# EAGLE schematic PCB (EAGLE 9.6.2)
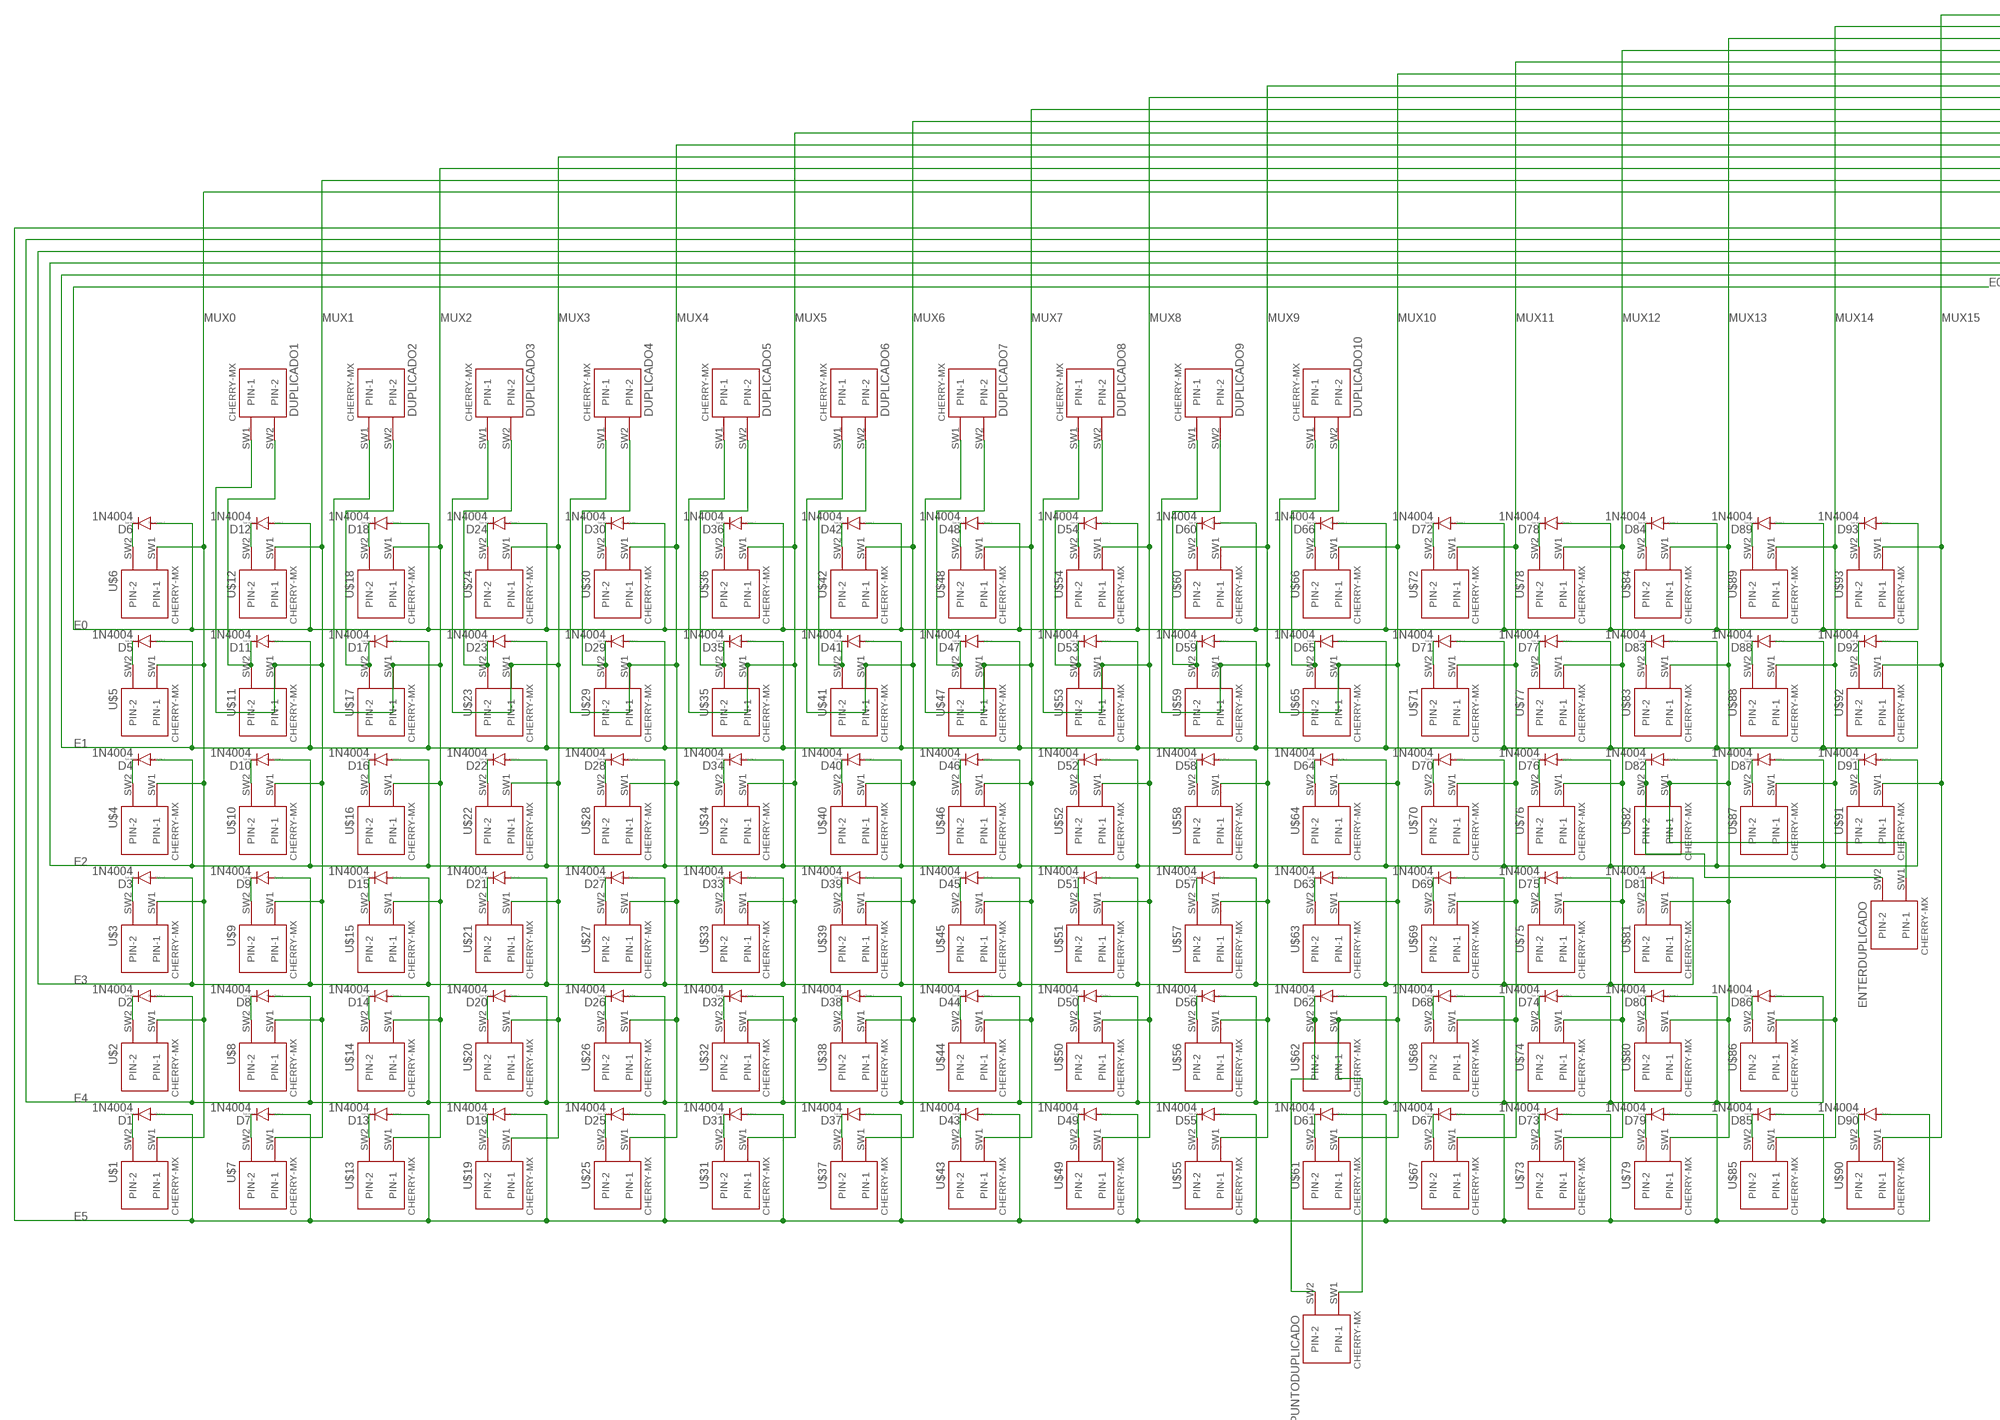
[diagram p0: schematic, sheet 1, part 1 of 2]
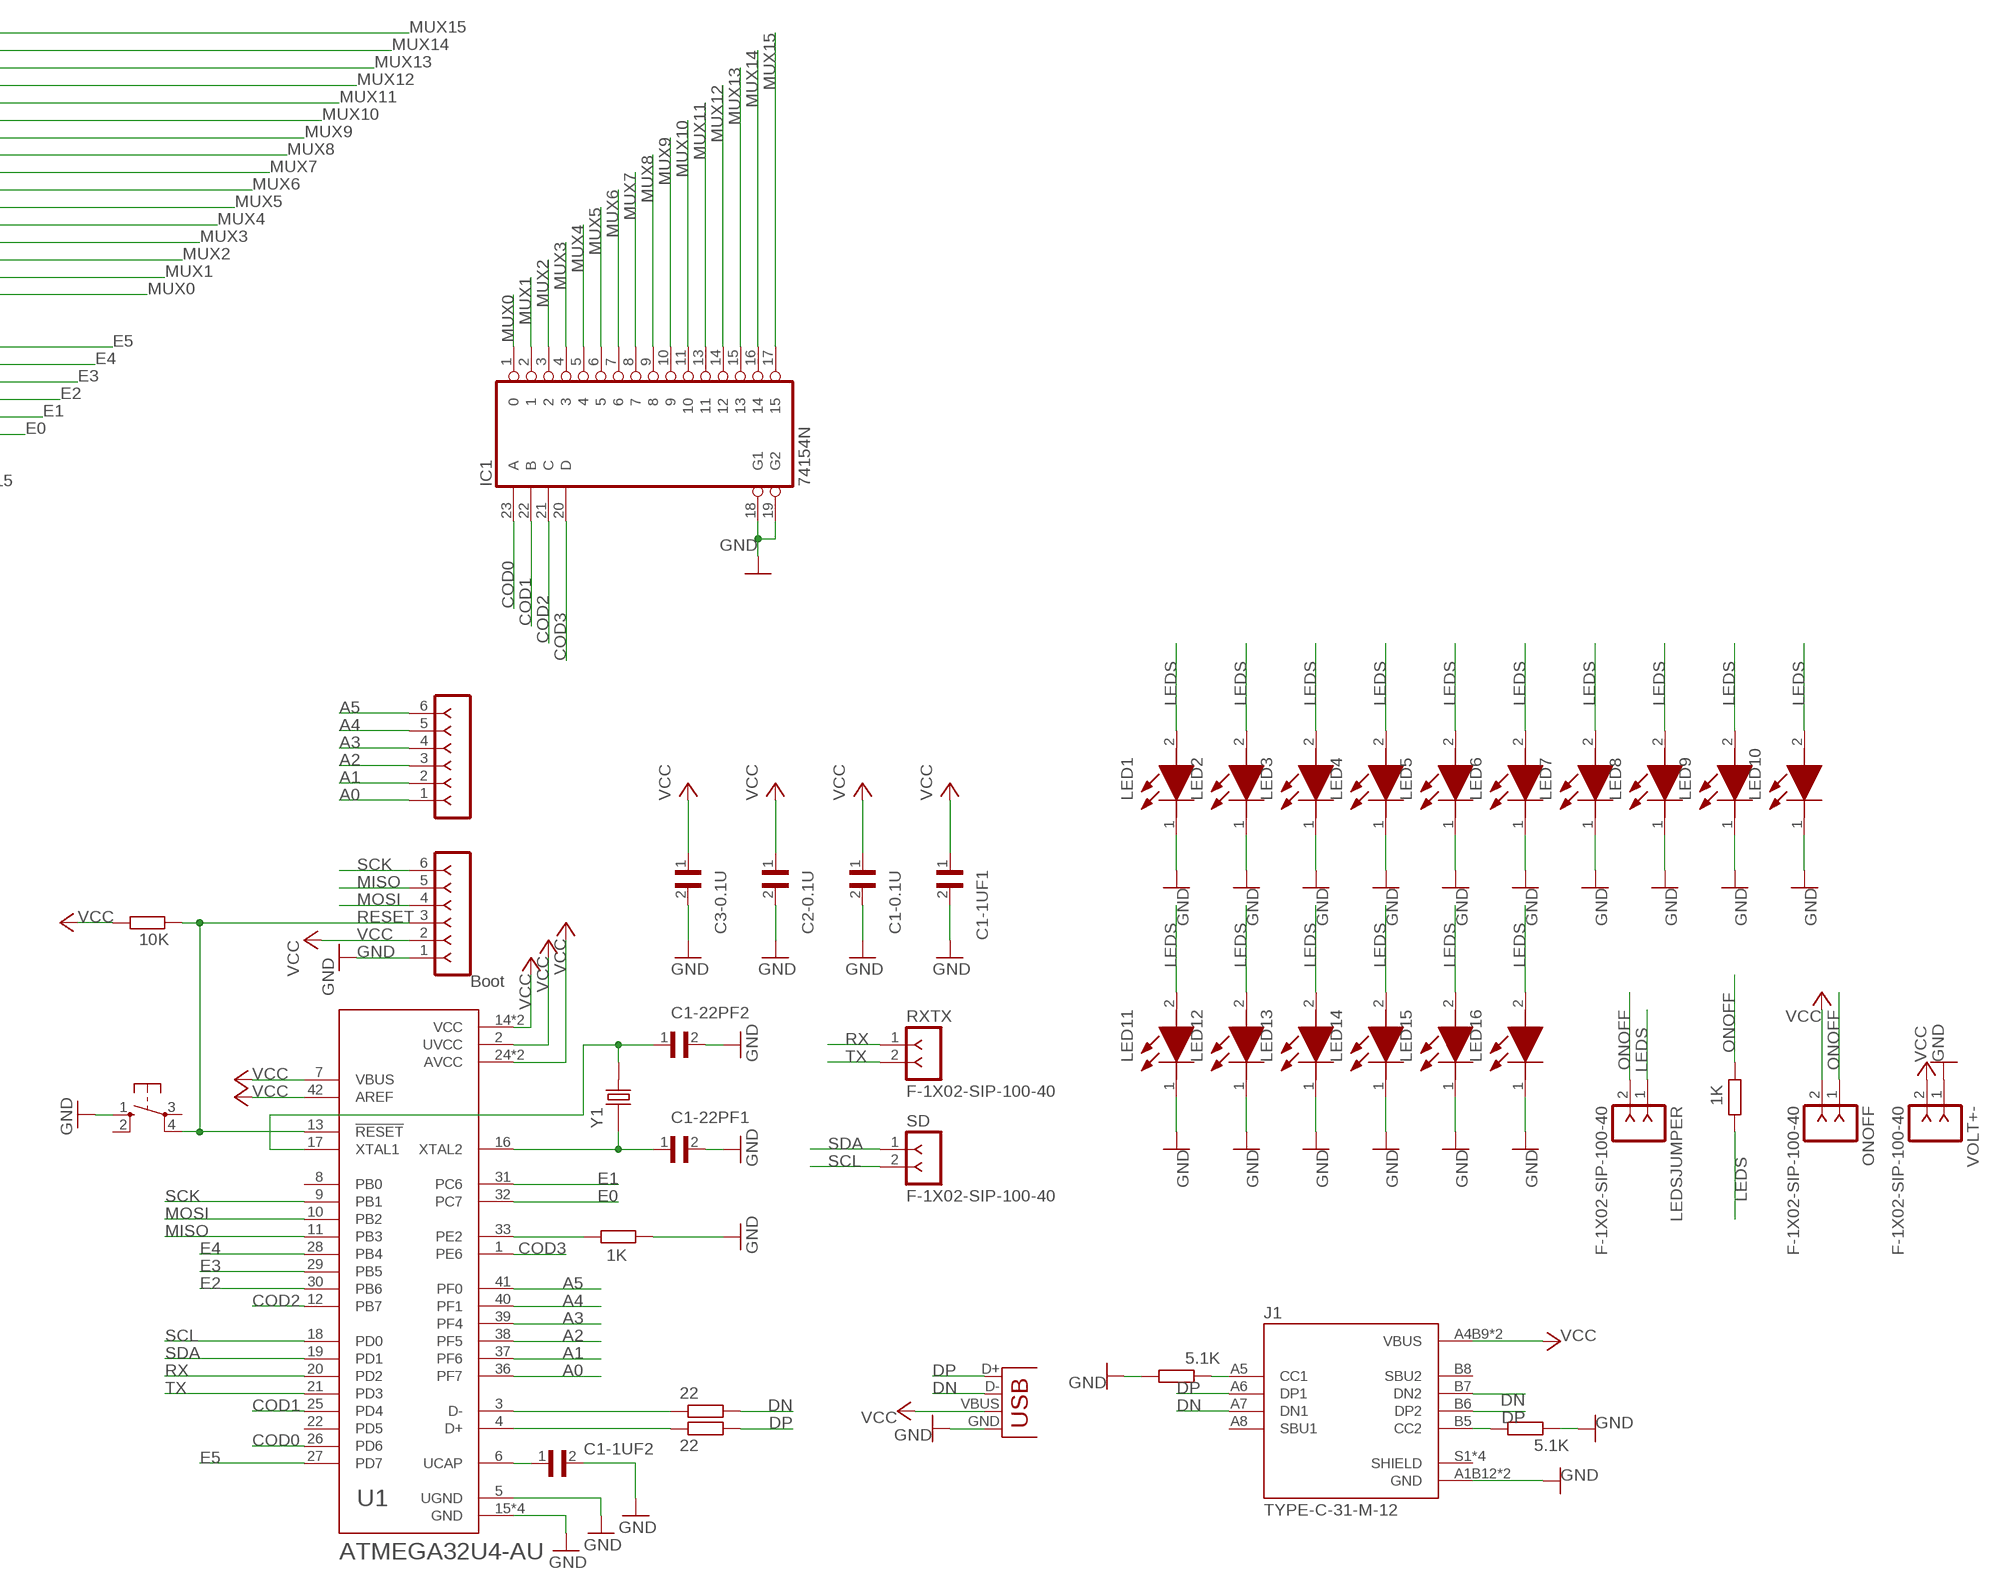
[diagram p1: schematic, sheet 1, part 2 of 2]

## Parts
ANALOG  Boot  F-1X06-SIP-100-32  [SIP-100-06-32]
BUTTON  10-XX  [B3F-10XX]
C1-0.1U  RDE5C1H273J2M1H03A  [CAP_RDE5C1H273J2M1H03A]
C1-1UF1  RDE5C1H273J2M1H03A  [CAP_RDE5C1H273J2M1H03A]
C1-1UF2  RDE5C1H273J2M1H03A  [CAP_RDE5C1H273J2M1H03A]
C1-22PF1  RDE5C1H273J2M1H03A  [CAP_RDE5C1H273J2M1H03A]
C1-22PF2  RDE5C1H273J2M1H03A  [CAP_RDE5C1H273J2M1H03A]
C2-0.1U  RDE5C1H273J2M1H03A  [CAP_RDE5C1H273J2M1H03A]
C3-0.1U  RDE5C1H273J2M1H03A  [CAP_RDE5C1H273J2M1H03A]
D1  1N4004  [DO41-10]
D2  1N4004  [DO41-10]
D3  1N4004  [DO41-10]
D4  1N4004  [DO41-10]
D5  1N4004  [DO41-10]
D6  1N4004  [DO41-10]
D7  1N4004  [DO41-10]
D8  1N4004  [DO41-10]
D9  1N4004  [DO41-10]
D10  1N4004  [DO41-10]
D11  1N4004  [DO41-10]
D12  1N4004  [DO41-10]
D13  1N4004  [DO41-10]
D14  1N4004  [DO41-10]
D15  1N4004  [DO41-10]
D16  1N4004  [DO41-10]
D17  1N4004  [DO41-10]
D18  1N4004  [DO41-10]
D19  1N4004  [DO41-10]
D20  1N4004  [DO41-10]
D21  1N4004  [DO41-10]
D22  1N4004  [DO41-10]
D23  1N4004  [DO41-10]
D24  1N4004  [DO41-10]
D25  1N4004  [DO41-10]
D26  1N4004  [DO41-10]
D27  1N4004  [DO41-10]
D28  1N4004  [DO41-10]
D29  1N4004  [DO41-10]
D30  1N4004  [DO41-10]
D31  1N4004  [DO41-10]
D32  1N4004  [DO41-10]
D33  1N4004  [DO41-10]
D34  1N4004  [DO41-10]
D35  1N4004  [DO41-10]
D36  1N4004  [DO41-10]
D37  1N4004  [DO41-10]
D38  1N4004  [DO41-10]
D39  1N4004  [DO41-10]
D40  1N4004  [DO41-10]
D41  1N4004  [DO41-10]
D42  1N4004  [DO41-10]
D43  1N4004  [DO41-10]
D44  1N4004  [DO41-10]
D45  1N4004  [DO41-10]
D46  1N4004  [DO41-10]
D47  1N4004  [DO41-10]
D48  1N4004  [DO41-10]
D49  1N4004  [DO41-10]
D50  1N4004  [DO41-10]
D51  1N4004  [DO41-10]
D52  1N4004  [DO41-10]
D53  1N4004  [DO41-10]
D54  1N4004  [DO41-10]
D55  1N4004  [DO41-10]
D56  1N4004  [DO41-10]
D57  1N4004  [DO41-10]
D58  1N4004  [DO41-10]
D59  1N4004  [DO41-10]
D60  1N4004  [DO41-10]
D61  1N4004  [DO41-10]
D62  1N4004  [DO41-10]
D63  1N4004  [DO41-10]
D64  1N4004  [DO41-10]
D65  1N4004  [DO41-10]
D66  1N4004  [DO41-10]
D67  1N4004  [DO41-10]
D68  1N4004  [DO41-10]
D69  1N4004  [DO41-10]
D70  1N4004  [DO41-10]
D71  1N4004  [DO41-10]
D72  1N4004  [DO41-10]
D73  1N4004  [DO41-10]
D74  1N4004  [DO41-10]
D75  1N4004  [DO41-10]
D76  1N4004  [DO41-10]
D77  1N4004  [DO41-10]
D78  1N4004  [DO41-10]
D79  1N4004  [DO41-10]
D80  1N4004  [DO41-10]
D81  1N4004  [DO41-10]
D82  1N4004  [DO41-10]
D83  1N4004  [DO41-10]
D84  1N4004  [DO41-10]
D85  1N4004  [DO41-10]
D86  1N4004  [DO41-10]
D87  1N4004  [DO41-10]
D88  1N4004  [DO41-10]
D89  1N4004  [DO41-10]
D90  1N4004  [DO41-10]
D91  1N4004  [DO41-10]
D92  1N4004  [DO41-10]
D93  1N4004  [DO41-10]
DUPLICADO1  CHERRY-MX  [CHERRY-MX]
DUPLICADO2  CHERRY-MX  [CHERRY-MX]
DUPLICADO3  CHERRY-MX  [CHERRY-MX]
DUPLICADO4  CHERRY-MX  [CHERRY-MX]
DUPLICADO5  CHERRY-MX  [CHERRY-MX]
DUPLICADO6  CHERRY-MX  [CHERRY-MX]
DUPLICADO7  CHERRY-MX  [CHERRY-MX]
DUPLICADO8  CHERRY-MX  [CHERRY-MX]
DUPLICADO9  CHERRY-MX  [CHERRY-MX]
DUPLICADO10  CHERRY-MX  [CHERRY-MX]
ENTERDUPLICADO  CHERRY-MX  [CHERRY-MX]
IC1  74154N  [DIL24-6]
J1  TYPE-C-31-M-12  [HRO_TYPE-C-31-M-12]
J3  Boot  F-1X06-SIP-100-32  [SIP-100-06-32]
LED1  ASMM-CA03-AS402  [LEDM3528X200N]
LED2  ASMM-CA03-AS402  [LEDM3528X200N]
LED3  ASMM-CA03-AS402  [LEDM3528X200N]
LED4  ASMM-CA03-AS402  [LEDM3528X200N]
LED5  ASMM-CA03-AS402  [LEDM3528X200N]
LED6  ASMM-CA03-AS402  [LEDM3528X200N]
LED7  ASMM-CA03-AS402  [LEDM3528X200N]
LED8  ASMM-CA03-AS402  [LEDM3528X200N]
LED9  ASMM-CA03-AS402  [LEDM3528X200N]
LED10  ASMM-CA03-AS402  [LEDM3528X200N]
LED11  ASMM-CA03-AS402  [LEDM3528X200N]
LED12  ASMM-CA03-AS402  [LEDM3528X200N]
LED13  ASMM-CA03-AS402  [LEDM3528X200N]
LED14  ASMM-CA03-AS402  [LEDM3528X200N]
LED15  ASMM-CA03-AS402  [LEDM3528X200N]
LED16  ASMM-CA03-AS402  [LEDM3528X200N]
LEDSJUMPER  F-1X02-SIP-100-40  [SIP-100-02-40]
ONOFF  F-1X02-SIP-100-40  [SIP-100-02-40]
PUNTODUPLICADO  CHERRY-MX  [CHERRY-MX]
R1  22  R-EU_0204/7  [0204/7]
R2  22  R-EU_0204/7  [0204/7]
R3  1K  R-EU_0204/7  [0204/7]
R4  1K  R-EU_0204/7  [0204/7]
R5  10K  R-EU_0204/7  [0204/7]
R6  5.1K  R-EU_0204/7  [0204/7]
R7  5.1K  R-EU_0204/7  [0204/7]
RXTX  F-1X02-SIP-100-40  [SIP-100-02-40]
SD  F-1X02-SIP-100-40  [SIP-100-02-40]
U1  ATMEGA32U4-AU  [QFP80P1200X1200X120-44N]
U$1  CHERRY-MX  [CHERRY-MX]
U$2  CHERRY-MX  [CHERRY-MX]
U$3  CHERRY-MX  [CHERRY-MX]
U$4  CHERRY-MX  [CHERRY-MX]
U$5  CHERRY-MX  [CHERRY-MX]
U$6  CHERRY-MX  [CHERRY-MX]
U$7  CHERRY-MX  [CHERRY-MX]
U$8  CHERRY-MX  [CHERRY-MX]
U$9  CHERRY-MX  [CHERRY-MX]
U$10  CHERRY-MX  [CHERRY-MX]
U$11  CHERRY-MX  [CHERRY-MX]
U$12  CHERRY-MX  [CHERRY-MX]
U$13  CHERRY-MX  [CHERRY-MX]
U$14  CHERRY-MX  [CHERRY-MX]
U$15  CHERRY-MX  [CHERRY-MX]
U$16  CHERRY-MX  [CHERRY-MX]
U$17  CHERRY-MX  [CHERRY-MX]
U$18  CHERRY-MX  [CHERRY-MX]
U$19  CHERRY-MX  [CHERRY-MX]
U$20  CHERRY-MX  [CHERRY-MX]
U$21  CHERRY-MX  [CHERRY-MX]
U$22  CHERRY-MX  [CHERRY-MX]
U$23  CHERRY-MX  [CHERRY-MX]
U$24  CHERRY-MX  [CHERRY-MX]
U$25  CHERRY-MX  [CHERRY-MX]
U$26  CHERRY-MX  [CHERRY-MX]
U$27  CHERRY-MX  [CHERRY-MX]
U$28  CHERRY-MX  [CHERRY-MX]
U$29  CHERRY-MX  [CHERRY-MX]
U$30  CHERRY-MX  [CHERRY-MX]
U$31  CHERRY-MX  [CHERRY-MX]
U$32  CHERRY-MX  [CHERRY-MX]
U$33  CHERRY-MX  [CHERRY-MX]
U$34  CHERRY-MX  [CHERRY-MX]
U$35  CHERRY-MX  [CHERRY-MX]
U$36  CHERRY-MX  [CHERRY-MX]
U$37  CHERRY-MX  [CHERRY-MX]
U$38  CHERRY-MX  [CHERRY-MX]
U$39  CHERRY-MX  [CHERRY-MX]
U$40  CHERRY-MX  [CHERRY-MX]
U$41  CHERRY-MX  [CHERRY-MX]
U$42  CHERRY-MX  [CHERRY-MX]
U$43  CHERRY-MX  [CHERRY-MX]
U$44  CHERRY-MX  [CHERRY-MX]
U$45  CHERRY-MX  [CHERRY-MX]
U$46  CHERRY-MX  [CHERRY-MX]
U$47  CHERRY-MX  [CHERRY-MX]
U$48  CHERRY-MX  [CHERRY-MX]
U$49  CHERRY-MX  [CHERRY-MX]
U$50  CHERRY-MX  [CHERRY-MX]
U$51  CHERRY-MX  [CHERRY-MX]
U$52  CHERRY-MX  [CHERRY-MX]
U$53  CHERRY-MX  [CHERRY-MX]
U$54  CHERRY-MX  [CHERRY-MX]
U$55  CHERRY-MX  [CHERRY-MX]
U$56  CHERRY-MX  [CHERRY-MX]
U$57  CHERRY-MX  [CHERRY-MX]
U$58  CHERRY-MX  [CHERRY-MX]
U$59  CHERRY-MX  [CHERRY-MX]
U$60  CHERRY-MX  [CHERRY-MX]
U$61  CHERRY-MX  [CHERRY-MX]
U$62  CHERRY-MX  [CHERRY-MX]
U$63  CHERRY-MX  [CHERRY-MX]
U$64  CHERRY-MX  [CHERRY-MX]
U$65  CHERRY-MX  [CHERRY-MX]
U$66  CHERRY-MX  [CHERRY-MX]
U$67  CHERRY-MX  [CHERRY-MX]
U$68  CHERRY-MX  [CHERRY-MX]
U$69  CHERRY-MX  [CHERRY-MX]
U$70  CHERRY-MX  [CHERRY-MX]
U$71  CHERRY-MX  [CHERRY-MX]
U$72  CHERRY-MX  [CHERRY-MX]
U$73  CHERRY-MX  [CHERRY-MX]
U$74  CHERRY-MX  [CHERRY-MX]
U$75  CHERRY-MX  [CHERRY-MX]
U$76  CHERRY-MX  [CHERRY-MX]
U$77  CHERRY-MX  [CHERRY-MX]
U$78  CHERRY-MX  [CHERRY-MX]
U$79  CHERRY-MX  [CHERRY-MX]
U$80  CHERRY-MX  [CHERRY-MX]
U$81  CHERRY-MX  [CHERRY-MX]
U$82  CHERRY-MX  [CHERRY-MX]
U$83  CHERRY-MX  [CHERRY-MX]
U$84  CHERRY-MX  [CHERRY-MX]
U$85  CHERRY-MX  [CHERRY-MX]
U$86  CHERRY-MX  [CHERRY-MX]
U$87  CHERRY-MX  [CHERRY-MX]
U$88  CHERRY-MX  [CHERRY-MX]
U$89  CHERRY-MX  [CHERRY-MX]
U$90  CHERRY-MX  [CHERRY-MX]
U$91  CHERRY-MX  [CHERRY-MX]
U$92  CHERRY-MX  [CHERRY-MX]
U$93  CHERRY-MX  [CHERRY-MX]
VOLT+-  F-1X02-SIP-100-40  [SIP-100-02-40]
X2  USB-A-H  [USB-A-H]
Y1  ECS-160-20-4X  [XTAL_ECS-160-20-4X]

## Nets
A0: ANALOG.1 U1.36(PF7)
A1: ANALOG.2 U1.37(PF6)
A2: ANALOG.3 U1.38(PF5)
A3: ANALOG.4 U1.39(PF4)
A4: ANALOG.5 U1.40(PF1)
A5: ANALOG.6 U1.41(PF0)
COD0: IC1.23(A) U1.26(PD6)
COD1: IC1.22(B) U1.25(PD4)
COD2: IC1.21(C) U1.12(PB7)
COD3: IC1.20(D) U1.1(PE6)
COMMON: J1.A5(CC1) R6.1
COMMON2: J1.B5(CC2) R7.1
D+: R1.1 U1.4(D+)
D-: R2.1 U1.3(D-)
DN: J1.A7(DN1) J1.B7(DN2) R2.2 X2.D-
DP: J1.A6(DP1) J1.B6(DP2) R1.2 X2.D+
E0: D6.A D12.A D18.A D24.A D30.A D36.A D42.A D48.A D54.A D60.A D66.A D72.A D78.A D84.A D89.A D93.A U1.32(PC7)
E1: D5.A D11.A D17.A D23.A D29.A D35.A D41.A D47.A D53.A D59.A D65.A D71.A D77.A D83.A D88.A D92.A U1.31(PC6)
E2: D4.A D10.A D16.A D22.A D28.A D34.A D40.A D46.A D52.A D58.A D64.A D70.A D76.A D82.A D87.A D91.A U1.30(PB6)
E3: D3.A D9.A D15.A D21.A D27.A D33.A D39.A D45.A D51.A D57.A D63.A D69.A D75.A D81.A U1.29(PB5)
E4: D2.A D8.A D14.A D20.A D26.A D32.A D38.A D44.A D50.A D56.A D62.A D68.A D74.A D80.A D86.A U1.28(PB4)
E5: D1.A D7.A D13.A D19.A D25.A D31.A D37.A D43.A D49.A D55.A D61.A D67.A D73.A D79.A D85.A D90.A U1.27(PD7)
GND [vcc]: BUTTON.1(S) C1-0.1U.2 C1-1UF1.2 C1-1UF2.2 C1-22PF1.2 C1-22PF2.2 C2-0.1U.2 C3-0.1U.2 IC1.18(G1) IC1.19(G2) J1.A1B12(GND) J1.B1A12(GND) J3.1 LED1.1(K) LED2.1(K) LED3.1(K) LED4.1(K) LED5.1(K) LED6.1(K) LED7.1(K) LED8.1(K) LED9.1(K) LED10.1(K) LED11.1(K) LED12.1(K) LED13.1(K) LED14.1(K) LED15.1(K) LED16.1(K) R4.1 R6.2 R7.2 U1.5(UGND) U1.15(GND) U1.23(GND) U1.35(GND) U1.43(GND) VOLT+-.1 X2.GND
LEDS: LED1.2(A) LED2.2(A) LED3.2(A) LED4.2(A) LED5.2(A) LED6.2(A) LED7.2(A) LED8.2(A) LED9.2(A) LED10.2(A) LED11.2(A) LED12.2(A) LED13.2(A) LED14.2(A) LED15.2(A) LED16.2(A) LEDSJUMPER.1 R3.1
MISO: J3.5 U1.11(PB3)
MOSI: J3.4 U1.10(PB2)
MUX0: IC1.1 U$1.SW1(PIN-1) U$2.SW1(PIN-1) U$3.SW1(PIN-1) U$4.SW1(PIN-1) U$5.SW1(PIN-1) U$6.SW1(PIN-1)
MUX1: DUPLICADO1.SW1(PIN-1) IC1.2 U$7.SW1(PIN-1) U$8.SW1(PIN-1) U$9.SW1(PIN-1) U$10.SW1(PIN-1) U$11.SW1(PIN-1) U$12.SW1(PIN-1)
MUX2: DUPLICADO2.SW1(PIN-1) IC1.3 U$13.SW1(PIN-1) U$14.SW1(PIN-1) U$15.SW1(PIN-1) U$16.SW1(PIN-1) U$17.SW1(PIN-1) U$18.SW1(PIN-1)
MUX3: DUPLICADO3.SW1(PIN-1) IC1.4 U$19.SW1(PIN-1) U$20.SW1(PIN-1) U$21.SW1(PIN-1) U$22.SW1(PIN-1) U$23.SW1(PIN-1) U$24.SW1(PIN-1)
MUX4: DUPLICADO4.SW1(PIN-1) IC1.5 U$25.SW1(PIN-1) U$26.SW1(PIN-1) U$27.SW1(PIN-1) U$28.SW1(PIN-1) U$29.SW1(PIN-1) U$30.SW1(PIN-1)
MUX5: DUPLICADO5.SW1(PIN-1) IC1.6 U$31.SW1(PIN-1) U$32.SW1(PIN-1) U$33.SW1(PIN-1) U$34.SW1(PIN-1) U$35.SW1(PIN-1) U$36.SW1(PIN-1)
MUX6: DUPLICADO6.SW1(PIN-1) IC1.7 U$37.SW1(PIN-1) U$38.SW1(PIN-1) U$39.SW1(PIN-1) U$40.SW1(PIN-1) U$41.SW1(PIN-1) U$42.SW1(PIN-1)
MUX7: DUPLICADO7.SW1(PIN-1) IC1.8 U$43.SW1(PIN-1) U$44.SW1(PIN-1) U$45.SW1(PIN-1) U$46.SW1(PIN-1) U$47.SW1(PIN-1) U$48.SW1(PIN-1)
MUX8: DUPLICADO8.SW1(PIN-1) IC1.9 U$49.SW1(PIN-1) U$50.SW1(PIN-1) U$51.SW1(PIN-1) U$52.SW1(PIN-1) U$53.SW1(PIN-1) U$54.SW1(PIN-1)
MUX9: DUPLICADO9.SW1(PIN-1) IC1.10 U$55.SW1(PIN-1) U$56.SW1(PIN-1) U$57.SW1(PIN-1) U$58.SW1(PIN-1) U$59.SW1(PIN-1) U$60.SW1(PIN-1)
MUX10: DUPLICADO10.SW1(PIN-1) IC1.11 PUNTODUPLICADO.SW1(PIN-1) U$61.SW1(PIN-1) U$62.SW1(PIN-1) U$63.SW1(PIN-1) U$64.SW1(PIN-1) U$65.SW1(PIN-1) U$66.SW1(PIN-1)
MUX11: IC1.13 U$67.SW1(PIN-1) U$68.SW1(PIN-1) U$69.SW1(PIN-1) U$70.SW1(PIN-1) U$71.SW1(PIN-1) U$72.SW1(PIN-1)
MUX12: IC1.14 U$73.SW1(PIN-1) U$74.SW1(PIN-1) U$75.SW1(PIN-1) U$76.SW1(PIN-1) U$77.SW1(PIN-1) U$78.SW1(PIN-1)
MUX13: ENTERDUPLICADO.SW1(PIN-1) IC1.15 U$79.SW1(PIN-1) U$80.SW1(PIN-1) U$81.SW1(PIN-1) U$82.SW1(PIN-1) U$83.SW1(PIN-1) U$84.SW1(PIN-1)
MUX14: IC1.16 U$85.SW1(PIN-1) U$86.SW1(PIN-1) U$87.SW1(PIN-1) U$88.SW1(PIN-1) U$89.SW1(PIN-1)
MUX15: IC1.17 U$90.SW1(PIN-1) U$91.SW1(PIN-1) U$92.SW1(PIN-1) U$93.SW1(PIN-1)
N$1: D4.C U$4.SW2(PIN-2)
N$2: D10.C U$10.SW2(PIN-2)
N$3: D16.C U$16.SW2(PIN-2)
N$4: D22.C U$22.SW2(PIN-2)
N$5: D5.C U$5.SW2(PIN-2)
N$6: D6.C U$6.SW2(PIN-2)
N$7: D28.C U$28.SW2(PIN-2)
N$8: D34.C U$34.SW2(PIN-2)
N$9: D40.C U$40.SW2(PIN-2)
N$10: D46.C U$46.SW2(PIN-2)
N$11: D11.C DUPLICADO1.SW2(PIN-2) U$11.SW2(PIN-2)
N$12: D12.C U$12.SW2(PIN-2)
N$13: D52.C U$52.SW2(PIN-2)
N$14: D58.C U$58.SW2(PIN-2)
N$15: D64.C U$64.SW2(PIN-2)
N$16: D70.C U$70.SW2(PIN-2)
N$17: D17.C DUPLICADO2.SW2(PIN-2) U$17.SW2(PIN-2)
N$18: D18.C U$18.SW2(PIN-2)
N$19: D76.C U$76.SW2(PIN-2)
N$20: D87.C U$87.SW2(PIN-2)
N$21: D91.C U$91.SW2(PIN-2)
N$22: D81.C U$81.SW2(PIN-2)
N$23: D23.C DUPLICADO3.SW2(PIN-2) U$23.SW2(PIN-2)
N$24: D24.C U$24.SW2(PIN-2)
N$25: D75.C U$75.SW2(PIN-2)
N$26: D69.C U$69.SW2(PIN-2)
N$27: D63.C U$63.SW2(PIN-2)
N$28: D57.C U$57.SW2(PIN-2)
N$29: D29.C DUPLICADO4.SW2(PIN-2) U$29.SW2(PIN-2)
N$30: D30.C U$30.SW2(PIN-2)
N$37: D51.C U$51.SW2(PIN-2)
N$38: D45.C U$45.SW2(PIN-2)
N$39: D39.C U$39.SW2(PIN-2)
N$40: D33.C U$33.SW2(PIN-2)
N$41: D35.C DUPLICADO5.SW2(PIN-2) U$35.SW2(PIN-2)
N$42: D36.C U$36.SW2(PIN-2)
N$43: D27.C U$27.SW2(PIN-2)
N$44: D21.C U$21.SW2(PIN-2)
N$45: D15.C U$15.SW2(PIN-2)
N$46: D9.C U$9.SW2(PIN-2)
N$47: D41.C DUPLICADO6.SW2(PIN-2) U$41.SW2(PIN-2)
N$48: D42.C U$42.SW2(PIN-2)
N$49: D3.C U$3.SW2(PIN-2)
N$50: D2.C U$2.SW2(PIN-2)
N$51: D8.C U$8.SW2(PIN-2)
N$52: D14.C U$14.SW2(PIN-2)
N$53: D47.C DUPLICADO7.SW2(PIN-2) U$47.SW2(PIN-2)
N$54: D48.C U$48.SW2(PIN-2)
N$55: D20.C U$20.SW2(PIN-2)
N$56: D26.C U$26.SW2(PIN-2)
N$57: D32.C U$32.SW2(PIN-2)
N$58: D38.C U$38.SW2(PIN-2)
N$59: D53.C DUPLICADO8.SW2(PIN-2) U$53.SW2(PIN-2)
N$60: D54.C U$54.SW2(PIN-2)
N$61: D44.C U$44.SW2(PIN-2)
N$62: D50.C U$50.SW2(PIN-2)
N$63: D56.C U$56.SW2(PIN-2)
N$64: D68.C U$68.SW2(PIN-2)
N$65: D59.C DUPLICADO9.SW2(PIN-2) U$59.SW2(PIN-2)
N$66: D60.C U$60.SW2(PIN-2)
N$67: D74.C U$74.SW2(PIN-2)
N$68: D62.C PUNTODUPLICADO.SW2(PIN-2) U$62.SW2(PIN-2)
N$69: D80.C U$80.SW2(PIN-2)
N$70: D86.C U$86.SW2(PIN-2)
N$71: D65.C DUPLICADO10.SW2(PIN-2) U$65.SW2(PIN-2)
N$72: D66.C U$66.SW2(PIN-2)
N$73: D90.C U$90.SW2(PIN-2)
N$74: D85.C U$85.SW2(PIN-2)
N$75: D79.C U$79.SW2(PIN-2)
N$76: D73.C U$73.SW2(PIN-2)
N$77: D71.C U$71.SW2(PIN-2)
N$78: D72.C U$72.SW2(PIN-2)
N$79: D67.C U$67.SW2(PIN-2)
N$80: D61.C U$61.SW2(PIN-2)
N$81: D55.C U$55.SW2(PIN-2)
N$82: D49.C U$49.SW2(PIN-2)
N$83: D77.C U$77.SW2(PIN-2)
N$84: D78.C U$78.SW2(PIN-2)
N$85: D43.C U$43.SW2(PIN-2)
N$86: D37.C U$37.SW2(PIN-2)
N$87: D31.C U$31.SW2(PIN-2)
N$88: D82.C ENTERDUPLICADO.SW2(PIN-2) U$82.SW2(PIN-2)
N$89: D83.C U$83.SW2(PIN-2)
N$90: D84.C U$84.SW2(PIN-2)
N$91: D25.C U$25.SW2(PIN-2)
N$92: D19.C U$19.SW2(PIN-2)
N$93: D13.C U$13.SW2(PIN-2)
N$94: D88.C U$88.SW2(PIN-2)
N$95: D89.C U$89.SW2(PIN-2)
N$96: D7.C U$7.SW2(PIN-2)
N$97: D1.C U$1.SW2(PIN-2)
N$98: D92.C U$92.SW2(PIN-2)
N$99: D93.C U$93.SW2(PIN-2)
ONOFF: LEDSJUMPER.2 ONOFF.1 R3.2
PE2: R4.2 U1.33(PE2)
RESET: BUTTON.4(P1) J3.3 R5.2 U1.13(!RESET)
RX: RXTX.1 U1.20(PD2)
SCK: J3.6 U1.9(PB1)
SCL: SD.2 U1.18(PD0)
SDA: SD.1 U1.19(PD1)
TX: RXTX.2 U1.21(PD3)
UCAP: C1-1UF2.1 U1.6(UCAP)
VCC: C1-0.1U.1 C1-1UF1.1 C2-0.1U.1 C3-0.1U.1 J1.A4B9(VBUS) J1.B4A9(VBUS) J3.2 ONOFF.2 R5.1 U1.2(UVCC) U1.7(VBUS) U1.14(VCC) U1.24(AVCC) U1.34(VCC) U1.42(AREF) U1.44(AVCC) VOLT+-.2 X2.VBUS
XTAL1: C1-22PF2.1 U1.17(XTAL1) Y1.2
XTAL2: C1-22PF1.1 U1.16(XTAL2) Y1.1
Unconnected: BUTTON.2(S1) BUTTON.3(P) J1.A8(SBU1) J1.B8(SBU2) J1.S1(SHIELD) J1.S2(SHIELD) J1.S3(SHIELD) J1.S4(SHIELD) U1.8(PB0) U1.22(PD5)

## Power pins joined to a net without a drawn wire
GND: IC1.12(GND)
VCC: IC1.24(VCC)

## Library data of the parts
ANALOG J3 = con-headers-jp:F-1X06-: FEMALE HEADER
BUTTON = switch-omron:10-XX: OMRON SWITCH; MPN: B3F-1000; OC_FARNELL: 176432; OC_NEWARK: 36M3542
C1-0.1U C1-1UF1 C1-1UF2 C1-22PF1 C1-22PF2 C2-0.1U C3-0.1U = Capacitor:RDE5C1H273J2M1H03A: Check prices; AVAILABILITY: In Stock; DESCRIPTION: Ceramic Capacitor; MF: Murata Electronics; MP: RDE5C1H273J2M1H03A; PACKAGE: NONSTANDARD; PRICE: None
D1-D93 = diode:1N4004: DIODE
DUPLICADO1-DUPLICADO10 ENTERDUPLICADO PUNTODUPLICADO U$1-U$93 = cherrymx:CHERRY-MX: Cherry MX series keyswitch
IC1 = 74_154:74*154: 4-line to 16-line data SELECTOR/MULTIPLEXER Check availability; AVAILABILITY: Not in stock; DESCRIPTION: 1 kOhms ±5% 0.063W, 1/16W Chip Resistor 0402 (1005 Metric) Thick Film; MF: TE Connectivity; MP: 74154; PACKAGE: None; PRICE: None
J1 = TYPE-C-31-M-12:TYPE-C-31-M-12: USB Connectors 24 Receptacle 1 8.94*7.3mm RoHS Check prices; AVAILABILITY: No availability data; DESCRIPTION: USB Connectors 24 Receptacle 1 8.94*7.3mm RoHS; MF: HRO Electronics Co., Ltd.; MP: TYPE-C-31-M-12; PACKAGE: Package; PRICE: None
LED1-LED16 = ASMM-CA03-AS402:ASMM-CA03-AS402: Standard LEDs - SMD PLCC2, SMD AlInGaP,Amber; DESCRIPTION: Standard LEDs - SMD PLCC2, SMD AlInGaP,Amber; HEIGHT: 2mm; MANUFACTURER_NAME: Avago Technologies; MANUFACTURER_PART_NUMBER: ASMM-CA03-AS402
LEDSJUMPER ONOFF RXTX SD VOLT+- = con-headers-jp:F-1X02-: FEMALE HEADER
R1-R7 = rcl:R-EU_: RESISTOR, European symbol; SPICEPREFIX: R
U1 = ATMEGA32U4-AU:ATMEGA32U4-AU: ATmega Series 16 MHz 32 KB Flash 2.5 KB SRAM 8-Bit Microcontroller - TQFP-44 Check prices; AVAILABILITY: Not in stock; DESCRIPTION: AVR AVR® ATmega Microcontroller IC 8-Bit 16MHz 32KB (16K x 16) FLASH 44-TQFP (10x10); MF: Microchip; MP: ATMEGA32U4-AU; PACKAGE: TQFP-44 Microchip; PRICE: None
X2 = con-usb:USB: USB Connectors
Y1 = Clock:ECS-160-20-4X: CRYSTAL T/H Check prices; AVAILABILITY: In Stock; DESCRIPTION: 16MHz ±30ppm Crystal 20pF 40 Ohms HC-49/US; MF: ECS Inc.; MP: ECS-160-20-4X; PACKAGE: HC-49US ECS Inc.; PRICE: None

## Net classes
0 default: width 0.203 mm

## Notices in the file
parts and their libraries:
con-headers-jp: Copyright (C) 2008, Bob Starr
